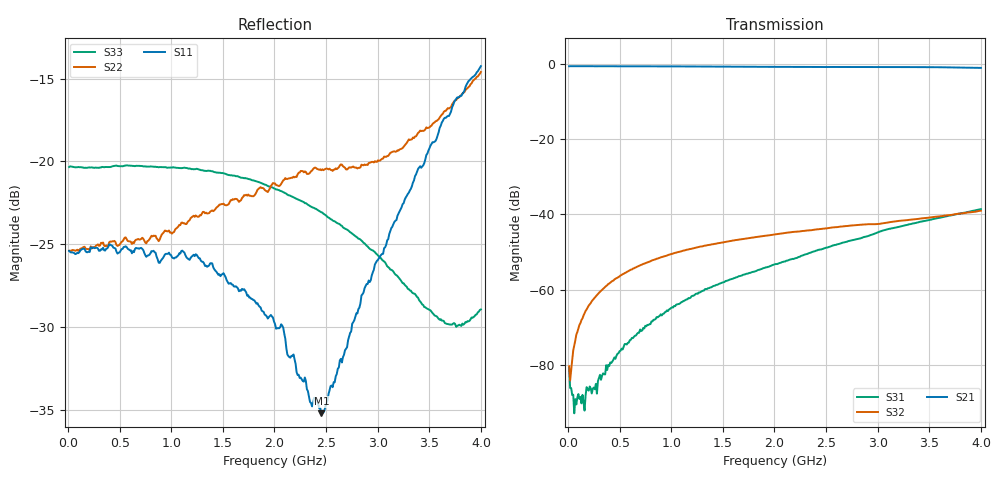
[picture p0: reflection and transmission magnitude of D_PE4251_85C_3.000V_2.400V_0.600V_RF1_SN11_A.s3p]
! Device ID: PE4251_SoldCshunt_081809
! Dir: c:\Test Bench Repositories\Bench_Software_CVI_Version_8\trunk\PSC 4Port_VNA Bench\datalog\4250\TEST\PE4251_SoldCshunt_081809\85C\3p000000\RF1
! Serial: 11
! Insertion: A
! Temp: 85C
! VDD: 3.000
! Control_Hi: 80.000
! Control_Lo: 20.000
! Logic State: RF1
! Port 1: RFC
! Port 2: RF1
! Port 3: RF2
! V1 = 0.60
! V2 = 2.40
! V3 = 0.60
! IDD: 5.307710e-05
! FILE NAME
! DATE 08/18/09  20:16
! CORRECTED  DATA
#  Hz  S  RI  R  50.00
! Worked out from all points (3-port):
!   401 points, 10 MHz to 4 GHz, reference 50 ohm
!   strongest paths, dB at 10 MHz, 1.008 GHz, 2.005 GHz, 3.002 GHz, 4 GHz:
!     S21: -0.6, -0.7, -0.8, -0.8, -1.1
!     S32: -80.4, -50.5, -45.3, -42.6, -39.0
!     S31: -80.7, -64.7, -53.2, -44.8, -38.6
!   lowest |S11| = -35.2 dB at 2.454 GHz (marker M1), VSWR 1.04, Z = 50 - j1.73 ohm
!   |S11| at or under -10 dB: start of sweep to end of sweep
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1e7  0.0536 -3.38e-05  0.93 -0.00393  -1.29e-05 -1.37e-05
     0.9295 -0.00411  0.0537 -2.73e-05  5.66e-05 7.77e-05
     9.19e-05 -4.7e-06  9.42e-05 -1.84e-05  0.0961 -0.000327
9.9775e7  0.0528 -0.00142  0.9315 -0.035  2.04e-05 -3.07e-05
          0.9309 -0.0352  0.0537 -0.00129  3.36e-05 0.000306
          3.23e-05 -2.53e-05  5.85e-05 0.0003  0.0961 -0.00239
1.79575e8  0.0532 -0.00139  0.9284 -0.0619  2.04e-06 -4.56e-05
           0.928 -0.0618  0.0544 -0.00146  5.33e-05 0.000543
           1.15e-05 -4.93e-05  7.51e-05 0.000541  0.0955 -0.00437
3.79075e8  0.0544 -0.00407  0.9206 -0.1266  -6.53e-05 -6.72e-05
           0.92 -0.1263  0.0553 -0.00317  0.000108 0.00115
           -6.3e-05 -5.8e-05  0.000109 0.00114  0.0956 -0.0098
5.0875e8  0.0533 -0.00614  0.912 -0.1692  -0.000119 -8.73e-05
          0.9124 -0.1687  0.0563 -0.00483  0.000159 0.00153
          -0.000131 -8.16e-05  0.000149 0.00154  0.0958 -0.0126
1.0474e9  0.0475 -0.0194  0.8614 -0.338  -0.000616 -8.7e-05
          0.8615 -0.337  0.0599 -0.0186  0.000467 0.00306
          -0.000625 -9.07e-05  0.000473 0.00306  0.0927 -0.0232
2.005e9  0.0264 -0.0185  0.7026 -0.582  -0.00215 0.000177
         0.7024 -0.5822  0.0722 -0.0463  0.000986 0.00533
         -0.00217 0.000178  0.000972 0.00533  0.0761 -0.0322
2.453875e9  1.68e-05 -0.0173  0.6105 -0.6727  -0.00341 0.000272
            0.6093 -0.6733  0.063 -0.0699  0.00103 0.0063
            -0.00341 0.000276  0.00102 0.00632  0.0617 -0.0335
3.670825e9  -0.1138 -0.0753  0.2763 -0.8563  -0.00898 0.00292
            0.279 -0.8548  -0.0642 -0.1285  -0.000149 0.00969
            -0.009 0.00289  -0.000134 0.00971  0.00418 -0.032
4e9  -0.176 -0.0811  0.1593 -0.8722  -0.0109 0.00447
     0.1581 -0.8697  -0.1363 -0.1269  -0.000787 0.0112
     -0.0109 0.00445  -0.000792 0.0112  -0.0158 -0.032
